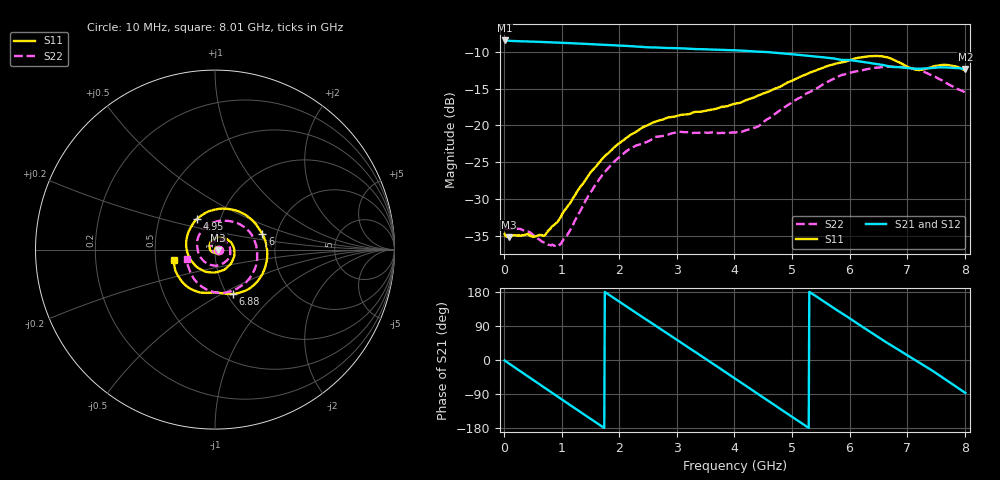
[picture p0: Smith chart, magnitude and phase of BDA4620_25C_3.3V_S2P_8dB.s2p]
!Agilent Technologies,E5071B,MY42404982,A.09.10
!Date: Wed May 06 08:50:04 2026
!Data & Calibration Information:
!Freq	S11:SOLT2(ON)	S21:SOLT2(ON)	S12:SOLT2(ON)	S22:SOLT2(ON)
# Hz S RI R 50
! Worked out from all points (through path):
!   801 points, 10 MHz to 8.01 GHz, reference 50 ohm
!   highest |S21| = -8.44 dB at 10 MHz (marker M1); lowest = -12.3 dB at 8.01 GHz (marker M2)
!   group delay of S21, straight-line fit = 280 ps
!   lowest |S11| = -35.2 dB at 80 MHz (marker M3), VSWR 1.04, Z = 51.7 - j0.338 ohm
!   |S11| at or under -10 dB: start of sweep to end of sweep
!   |S22| runs from -36.4 to -12.0 dB; largest |S21 - S12| = 0.0016
!   S11 on the Smith chart (normalised r, x): 10 MHz: 1.04, -0.00; 4.95 GHz: 0.77, +0.27; 6 GHz: 1.68, +0.31; 6.88 GHz: 1.06, -0.57; 8.01 GHz: 0.63, -0.08
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1e7  0.0183 -0.00136  0.3782 -0.0083  0.3789 -0.00824  0.0203 -0.00122
8e7  0.0172 -0.00327  0.3722 -0.0568  0.3725 -0.0571  0.0195 -0.00272
4.4e8  0.00947 -0.0152  0.2581 -0.2676  0.2587 -0.2679  0.0134 -0.0132
7.4e8  -0.00776 -0.0169  0.0827 -0.3589  0.0826 -0.3595  -0.000515 -0.0156
9.7e8  -0.022 -0.00802  -0.0679 -0.359  -0.068 -0.3593  -0.0126 -0.009
1.35e9  -0.0303 0.0251  -0.2743 -0.2326  -0.2746 -0.2328  -0.0213 0.0172
1.65e9  -0.0126 0.0544  -0.3494 -0.0599  -0.35 -0.0599  -0.0099 0.0416
1.94e9  0.0224 0.069  -0.3293 0.1183  -0.3299 0.1187  0.017 0.0556
2.32e9  0.0759 0.0518  -0.18 0.2925  -0.1806 0.2932  0.0589 0.0442
2.68e9  0.1078 -0.00158  0.0258 0.3373  0.0265 0.3376  0.0835 0.00812
3e9  0.097 -0.0635  0.2 0.269  0.2005 0.2693  0.0827 -0.0356
3.39e9  0.0369 -0.1181  0.3204 0.0806  0.3211 0.0803  0.0417 -0.0787
4.01e9  -0.1051 -0.0931  0.2128 -0.2443  0.2131 -0.2448  -0.0633 -0.0637
4.48e9  -0.1612 0.0287  -0.0376 -0.3149  -0.0376 -0.3154  -0.1001 0.0258
4.95e9  -0.1019 0.1694  -0.2502 -0.1764  -0.2506 -0.1765  -0.046 0.1315
5.35e9  0.0391 0.2287  -0.294 0.0265  -0.2942 0.0267  0.0626 0.1602
6e9  0.2637 0.0865  -0.095 0.2613  -0.0952 0.2617  0.2233 0.0422
6.34e9  0.285 -0.0779  0.0652 0.2586  0.0657 0.2588  0.232 -0.0725
6.68e9  0.186 -0.2203  0.1856 0.1707  0.1863 0.1708  0.1751 -0.1804
6.88e9  0.0989 -0.2473  0.2271 0.1013  0.2277 0.1016  0.1167 -0.2207
7.44e9  -0.0723 -0.2402  0.2161 -0.1174  0.2166 -0.1178  -0.0771 -0.2042
8.01e9  -0.2277 -0.0586  0.0135 -0.2412  0.0134 -0.2418  -0.1585 -0.0521
